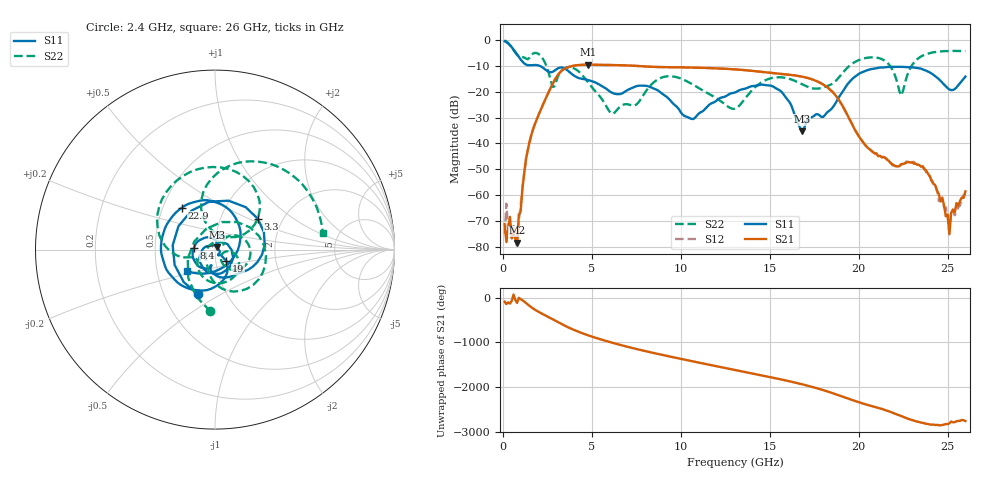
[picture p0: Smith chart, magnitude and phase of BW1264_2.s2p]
!Keysight Technologies,N5245B,MY57181159,A.13.60.06
!Date: Friday, December 18, 2020 23:52:02
!Correction: S11(Full 2 Port(1,2))
!S21(Full 2 Port(1,2))
!S12(Full 2 Port(1,2))
!S22(Full 2 Port(1,2))
!S2P File: Measurements: S11, S21, S12, S22:
# Hz S  dB  R 50
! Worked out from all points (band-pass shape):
!   260 points, 100 MHz to 26 GHz, reference 50 ohm
!   highest |S21| = -9.56 dB at 4.8 GHz (marker M1); lowest = -78.4 dB at 800 MHz (marker M2)
!   |S21| within 3 dB of the highest: 3.207 GHz to 14.81 GHz (11.61 GHz wide, 129 % of centre)
!   lowest |S11| = -35.3 dB at 16.8 GHz (marker M3), VSWR 1.03, Z = 51.1 + j1.36 ohm
!   |S11| at or under -10 dB: 2.06 GHz to end of sweep
!   |S22| runs from -28.5 to -0.2 dB; largest |S21 - S12| = 0.00077
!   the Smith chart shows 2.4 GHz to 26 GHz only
!   S11 on the Smith chart (normalised r, x): 2.4 GHz: 0.74, -0.40; 3.3 GHz: 1.50, +0.56; 8.4 GHz: 0.79, +0.01; 19 GHz: 1.12, -0.14; 22.9 GHz: 0.63, +0.32; 26 GHz: 0.72, -0.18
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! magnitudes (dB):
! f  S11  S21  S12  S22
! 100 MHz  -0.5  -71.2  -75.0  -0.2
! 200 MHz  -0.8  -78.1  -63.3  -0.6
! 800 MHz  -5.6  -78.4  -79.7  -5.8
! 1.4 GHz  -9.7  -42.6  -42.6  -7.5
! 2.4 GHz  -11.5  -22.8  -22.8  -9.2
! 3.3 GHz  -10.6  -11.9  -11.9  -11.8
! 4.5 GHz  -15.1  -9.6  -9.6  -13.9
! 4.8 GHz  -15.5  -9.6  -9.6  -16.5
! 6.2 GHz  -20.6  -9.7  -9.7  -28.5
! 8.4 GHz  -18.5  -10.4  -10.4  -16.9
! 8.8 GHz  -19.9  -10.5  -10.5  -14.9
! 10.7 GHz  -30.6  -10.7  -10.7  -17.3
! 13.1 GHz  -20.2  -11.4  -11.4  -26.4
! 15.5 GHz  -19.2  -13.0  -13.0  -14.4
! 16.8 GHz  -35.3  -14.2  -14.2  -17.1
! 17.4 GHz  -29.7  -15.3  -15.3  -18.7
! 19 GHz  -21.0  -24.4  -24.4  -13.6
! 21.7 GHz  -10.4  -46.8  -46.5  -9.5
! 22.4 GHz  -10.4  -48.0  -48.0  -21.4
! 22.9 GHz  -10.5  -47.4  -47.3  -10.9
! 25.1 GHz  -19.1  -75.1  -74.0  -4.3
! 26 GHz  -14.2  -58.5  -59.4  -4.3
